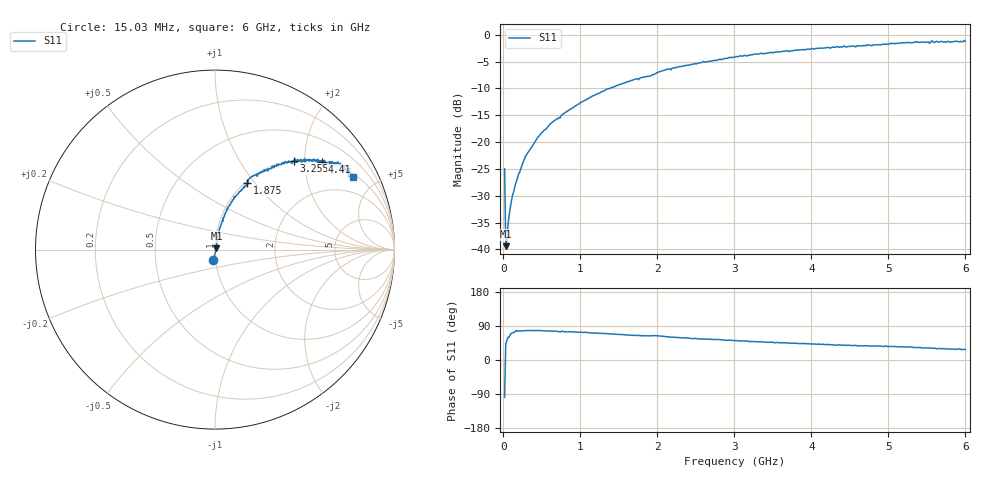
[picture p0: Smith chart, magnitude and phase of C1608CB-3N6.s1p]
!	Network	Analyzer	HP8753E.07.74:	Oct	30	2002	Serial	No.	JP38451487
!	Hewlett-Packard
!	27	Aug	2009	15:19:33
!	Frequency	S11
#	HZ	S	RI	R	50
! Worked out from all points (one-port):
!   400 points, 15.03 MHz to 6 GHz, reference 50 ohm
!   lowest |S11| = -39.4 dB at 30.03 MHz (marker M1), VSWR 1.02, Z = 50.8 + j0.74 ohm
!   |S11| at or under -10 dB: start of sweep to 1.382 GHz
!   S11 on the Smith chart (normalised r, x): 15.03 MHz: 0.98, -0.11; 1.875 GHz: 1.03, +0.91; 3.255 GHz: 1.00, +1.77; 4.41 GHz: 1.01, +2.44; 6 GHz: 1.13, +3.73
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1.502992e7  -0.00853 -0.0557
3.002985e7  0.00785 0.00728
4.502978e7  0.00755 0.00938
6.00297e7  0.00855 0.015
7.502962e7  0.0103 0.0182
1.200294e8  0.00975 0.0308
1.95029e8  0.0115 0.0488
2.850286e8  0.0157 0.072
4.950275e8  0.0257 0.12
7.650262e8  0.0437 0.175
1.155024e9  0.0868 0.254
1.515022e9  0.133 0.317
1.875021e9  0.18 0.369
2.265019e9  0.254 0.433
3.015015e9  0.391 0.491
3.255014e9  0.439 0.495
3.765011e9  0.507 0.497
4.410008e9  0.598 0.488
4.515007e9  0.612 0.482
5.265004e9  0.701 0.473
5.445003e9  0.732 0.447
5.520002e9  0.731 0.447
5.535002e9  0.706 0.437
5.565002e9  0.755 0.451
5.595002e9  0.721 0.443
5.625002e9  0.758 0.428
5.655002e9  0.736 0.432
6e9  0.769 0.404
